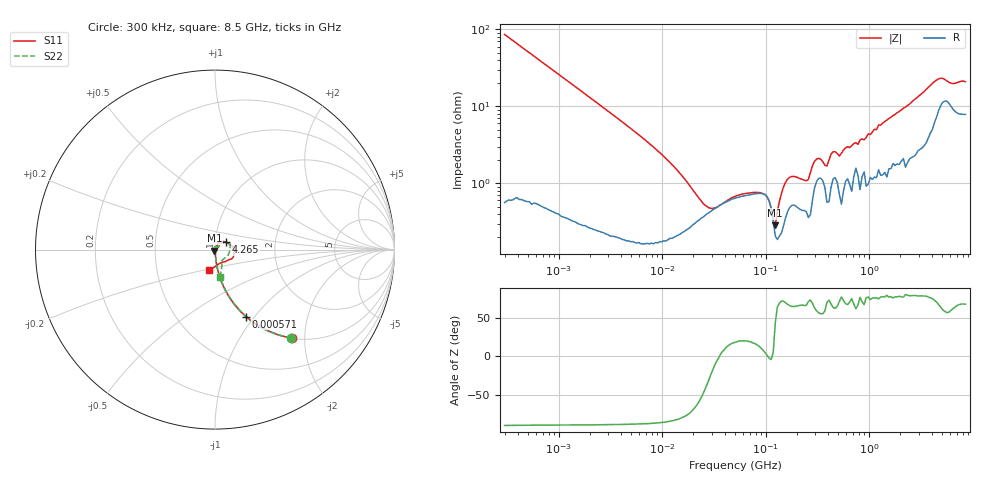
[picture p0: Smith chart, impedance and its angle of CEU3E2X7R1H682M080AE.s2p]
! S-parameter Generated by TDK Corporation
! Copyright(C) 2015 TDK Corporation.
! All Rights Reserved.
! TDK P/N: CEU3E2X7R1H682M080AE (Multilayer Ceramic Chip Capacitors)
! Property: C=6.8nF
! Size(LxWxT): 1.6x0.8x0.8mm, 0.063x0.031x0.031inches
! Model Type: s2p (Touchstone File Format Version 1.0)
! Frequency: DC=Yes Start=0.3MHz Stop=8500MHz 225points Log-sweep
! Note:
! Model Generated on Jun. 23, 2015
! Hash(MD5):
! Port Assignments:
!  1 ---| |--- 2
! Applicable Conditions:
!  Temperature = 25 degC
!  DC Bias Voltage = 0 V
!  Small Signal Operation
! Terms and conditions regarding TDK Simulation Models
! (1)This simulation model is being provided solely for informational purposes. Please refer to the specifications of the products in terms of detailed characteristics of such products.
! (2)In no event shall TDK Corporation of any of its subsidiaries be liable for any loss or damage arising, directly or indirectly,
!  From any information contained in this simulation model, including, but not limited to loss or damages arising from any inaccuracies, omissions or errors in connection with such information.
! (3)Any and all copyrights on this simulation model are owned by TDK Corporation.
!  Duplication or redistribution of this simulation model without prior written permission from TDK Corporation is prohibited.
! (4)This simulation model is subject to any modification or change without any prior notice.
! (5)Neither TDK Corporation nor any of its subsidiaries shall make any warranty, express or implied,
!  Including but not limited to the correctness, implied warranties of merchantability and fitness for a particular purpose with respect to this simulation models.
! (6)The use of this simulation model shall be deemed to have consented to the terms and conditions hereof.
# MHz S MA R 50
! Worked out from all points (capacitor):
!   224 points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, 300 kHz to 8.5 GHz, reference 50 ohm
!   read as one part in series: C = 6.15 nF near 314.1 kHz
!   lowest |Z| = 286 mohm at 123.8 MHz (marker M1)
!   series resonance near 35.63 MHz, so ESL is about 3.2 nH
!   S11 on the Smith chart (normalised r, x): 300 kHz: 1.01, -1.72; 571 kHz: 1.01, -0.91; 4.265 GHz: 1.13, +0.10; 8.5 GHz: 0.92, -0.21
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0.3  0.6512 -49.1  0.7553 40.5  0.7566 40.7  0.6498 -49.2
0.5710021  0.4115 -65.1  0.9059 24.3  0.9063 24.3  0.4112 -65.0
1.72111  0.1496 -80.4  0.9859 8.6  0.9861 8.6  0.1495 -80.4
9.430415  0.0255 -86.1  0.9976 1.4  0.998 1.4  0.02546 -84.0
24.76313  0.004721 -83.7  0.9957 0.1  0.996 0.2  0.008493 -46.8
35.77084  0.0003454 -130.1  0.9935 -0.2  0.9939 -0.1  0.009168 -26.8
51.67171  0.002532 129.9  0.9909 -0.4  0.9911 -0.3  0.01079 -28.7
123.7646  0.006024 -121.0  0.992 -0.5  0.9922 -0.5  0.006715 -132.3
283.1228  0.005217 -101.0  0.9848 -1.7  0.9854 -1.7  0.01136 113.3
373.0505  0.002142 -98.2  0.9824 -1.8  0.9827 -1.8  0.001328 -80.5
428.2171  0.002067 -28.0  0.9838 -2.4  0.9843 -2.3  0.008763 75.1
564.2308  0.005921 -133.3  0.9801 -2.9  0.9809 -2.9  0.00791 113.6
618.5683  0.001322 -17.9  0.9774 -3.0  0.9781 -3.0  0.006728 90.7
743.4462  0.009525 -44.7  0.9765 -3.3  0.9773 -3.3  0.01385 47.2
815.0429  0.001512 119.1  0.9836 -3.7  0.984 -3.7  0.01149 78.9
979.5854  0.001978 106.9  0.983 -4.7  0.9839 -4.6  0.00948 42.7
1232.735  0.01288 16.7  0.9793 -5.8  0.9797 -5.8  0.01696 61.2
1290.729  0.01161 63.0  0.977 -6.0  0.9775 -6.0  0.001737 52.2
1351.452  0.009907 14.0  0.9779 -6.2  0.9785 -6.2  0.01648 90.0
1551.304  0.01392 36.5  0.9744 -7.2  0.9752 -7.2  0.0109 77.7
4265.177  0.07545 35.4  0.9242 -19.4  0.925 -19.5  0.07512 33.4
8500  0.1185 -105.5  0.898 -31.1  0.8985 -31.2  0.1528 -79.7
